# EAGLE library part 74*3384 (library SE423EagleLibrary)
10-bit FET bus switches with level shifting
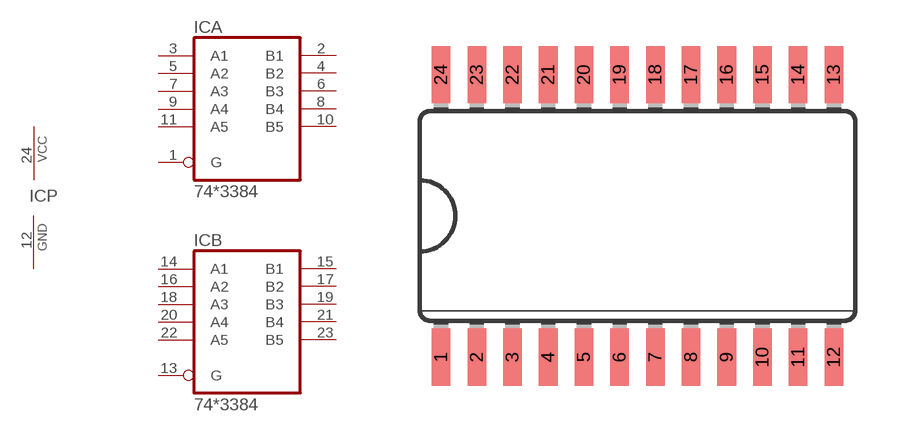
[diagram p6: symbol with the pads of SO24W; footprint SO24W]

Designator prefix IC; gates A=743384 B=743384 P=PWRN

## 743384DW  [SO24W]
1  A:G  in
2  A:B1
3  A:A1
4  A:B2
5  A:A2
6  A:B3
7  A:A3
8  A:B4
9  A:A4
10  A:B5
11  A:A5
12  P:GND  pwr
13  B:G  in
14  B:A1
15  B:B1
16  B:A2
17  B:B2
18  B:A3
19  B:B3
20  B:A4
21  B:B4
22  B:A5
23  B:B5
24  P:VCC  pwr

## Footprint SO24W (pad centres in mm)
Small Outline Package 24 wide
smd 0.66 x 2.032: 1 -6.985,-5.029; 2 -5.715,-5.029; 3 -4.445,-5.029; 4 -3.175,-5.029; 5 -1.905,-5.029; 6 -0.635,-5.029; 7 0.635,-5.029; 8 1.905,-5.029; 9 3.175,-5.029; 10 4.445,-5.029; 11 5.715,-5.029; 12 6.985,-5.029; 13 6.985,5.029; 14 5.715,5.029; 15 4.445,5.029; 16 3.175,5.029; 17 1.905,5.029; 18 0.635,5.029; 19 -0.635,5.029; 20 -1.905,5.029; 21 -3.175,5.029; 22 -4.445,5.029; 23 -5.715,5.029; 24 -6.985,5.029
